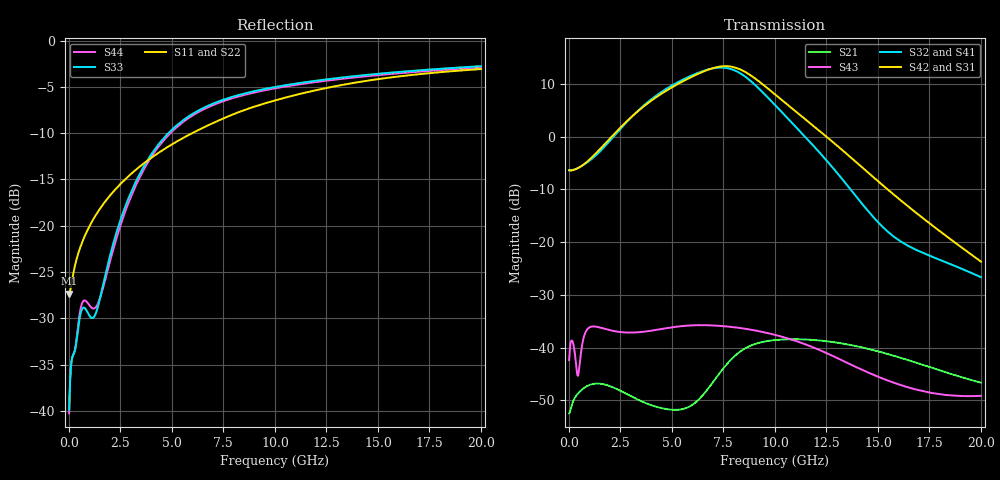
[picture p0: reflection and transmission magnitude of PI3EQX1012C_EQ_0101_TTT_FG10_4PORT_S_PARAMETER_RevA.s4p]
! NPort=4 DATA=2000 NOISE=0 GROUPDELAY=0 COMPLEX_DATAFORMAT=POLAR
! NumOfBlock=1 NumOfParam=0
! .MODEL Smodel S TSTONEFILE=PI3EQX1012C_EQ_0101_TTT_FG10_4PORT_S_PARAMETER_RevA.s4p TYPE=S
!  -- The above .MODEL line can be used for the S element in the netlist.
! The s parameter is extracted from the linear redriver, it is not bi-directional; only s(4,1)s(4,2) and s(3,1)s(3,2)
! should be the insertion loss
!Port definition:
!Port1 = input+
!Port2 = input-
!Port3 = output+
!Port4 = output-
# Hz S MA R  50
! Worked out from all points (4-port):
!   2000 points, 10 MHz to 20 GHz, reference 50 ohm
!   strongest paths, dB at 10 MHz, 5.01 GHz, 10.01 GHz, 15.01 GHz, 20 GHz:
!     S42: -6.4, 9.4, 8.0, -8.5, -23.7
!     S31: -6.4, 9.3, 7.9, -8.7, -24.1
!     S32: -6.4, 9.7, 6.0, -16.2, -26.6
!     S41: -6.4, 9.7, 6.1, -16.4, -27.0
!     S43: -42.4, -36.1, -37.6, -45.5, -49.1
!     S21: -52.4, -51.8, -38.6, -40.7, -46.6
!   lowest |S11| = -27.3 dB at 10 MHz (marker M1), VSWR 1.09, Z = 45.9 - j0.123 ohm
!   |S11| at or under -10 dB: start of sweep to 5.987 GHz
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1e7  0.04301 -178.2  0.002379 1.5  0.0008102 -0.5  0.0008039 -0.5
     0.002388 1.5  0.04109 -178.1  0.000927 -0.5  0.0009197 -0.5
     0.4784 -0.1  0.4775 179.9  0.01016 -4.0  0.007598 -25.7
     0.4771 179.9  0.4794 -0.2  0.007615 -25.8  0.009722 -4.0
4.12e9  0.2378 -124.3  0.002831 0.2  0.0003796 -56.9  0.0003778 -57.3
        0.002798 0.4  0.2415 -123.2  0.0004314 -57.6  0.0004294 -58.0
        2.276 -64.4  2.349 126.8  0.2543 -83.8  0.01363 33.4
        2.334 127.5  2.276 -62.7  0.01461 30.4  0.2464 -83.5
5.78e9  0.3076 -123.8  0.002778 35.0  0.0002761 -58.3  0.0002749 -59.3
        0.002723 33.6  0.3127 -123.2  0.0003129 -59.3  0.0003117 -60.2
        3.518 -130.9  3.655 59.9  0.3873 -99.7  0.01641 9.0
        3.665 60.1  3.536 -129.0  0.01619 6.3  0.3795 -99.5
7.09e9  0.3625 -124.5  0.005226 55.6  0.0002385 -55.8  0.0002364 -57.2
        0.004999 56.0  0.368 -124.0  0.0002689 -57.0  0.0002667 -58.4
        4.474 166.0  4.464 -3.8  0.4608 -109.8  0.01668 -11.3
        4.497 -3.9  4.505 168.2  0.0162 -12.5  0.4526 -109.7
8.24e9  0.4104 -125.9  0.009207 41.2  0.0002229 -54.2  0.0002198 -55.7
        0.008952 42.5  0.4164 -125.5  0.0002497 -55.4  0.0002463 -57.0
        4.356 101.1  4.06 -68.7  0.5078 -116.6  0.01578 -27.0
        4.104 -69.2  4.39 103.4  0.01542 -27.5  0.4993 -116.4
9.63e9  0.4619 -128.2  0.0117 13.7  0.0002131 -53.9  0.000209 -55.5
        0.01155 15.0  0.4689 -127.8  0.0002371 -55.1  0.0002327 -56.6
        2.86 30.7  2.376 -137.3  0.551 -122.8  0.01407 -43.5
        2.41 -138.3  2.884 33.4  0.01377 -44.0  0.5422 -122.7
2e10  0.7015 -144.6  0.004723 -69.0  0.0001465 -72.3  0.0001414 -73.8
      0.004662 -68.3  0.7165 -144.4  0.0001625 -72.1  0.0001567 -73.7
      0.06227 106.7  0.04654 33.6  0.7272 -143.5  0.003574 -51.6
      0.04488 31.9  0.06546 111.5  0.003493 -48.9  0.7152 -143.3
